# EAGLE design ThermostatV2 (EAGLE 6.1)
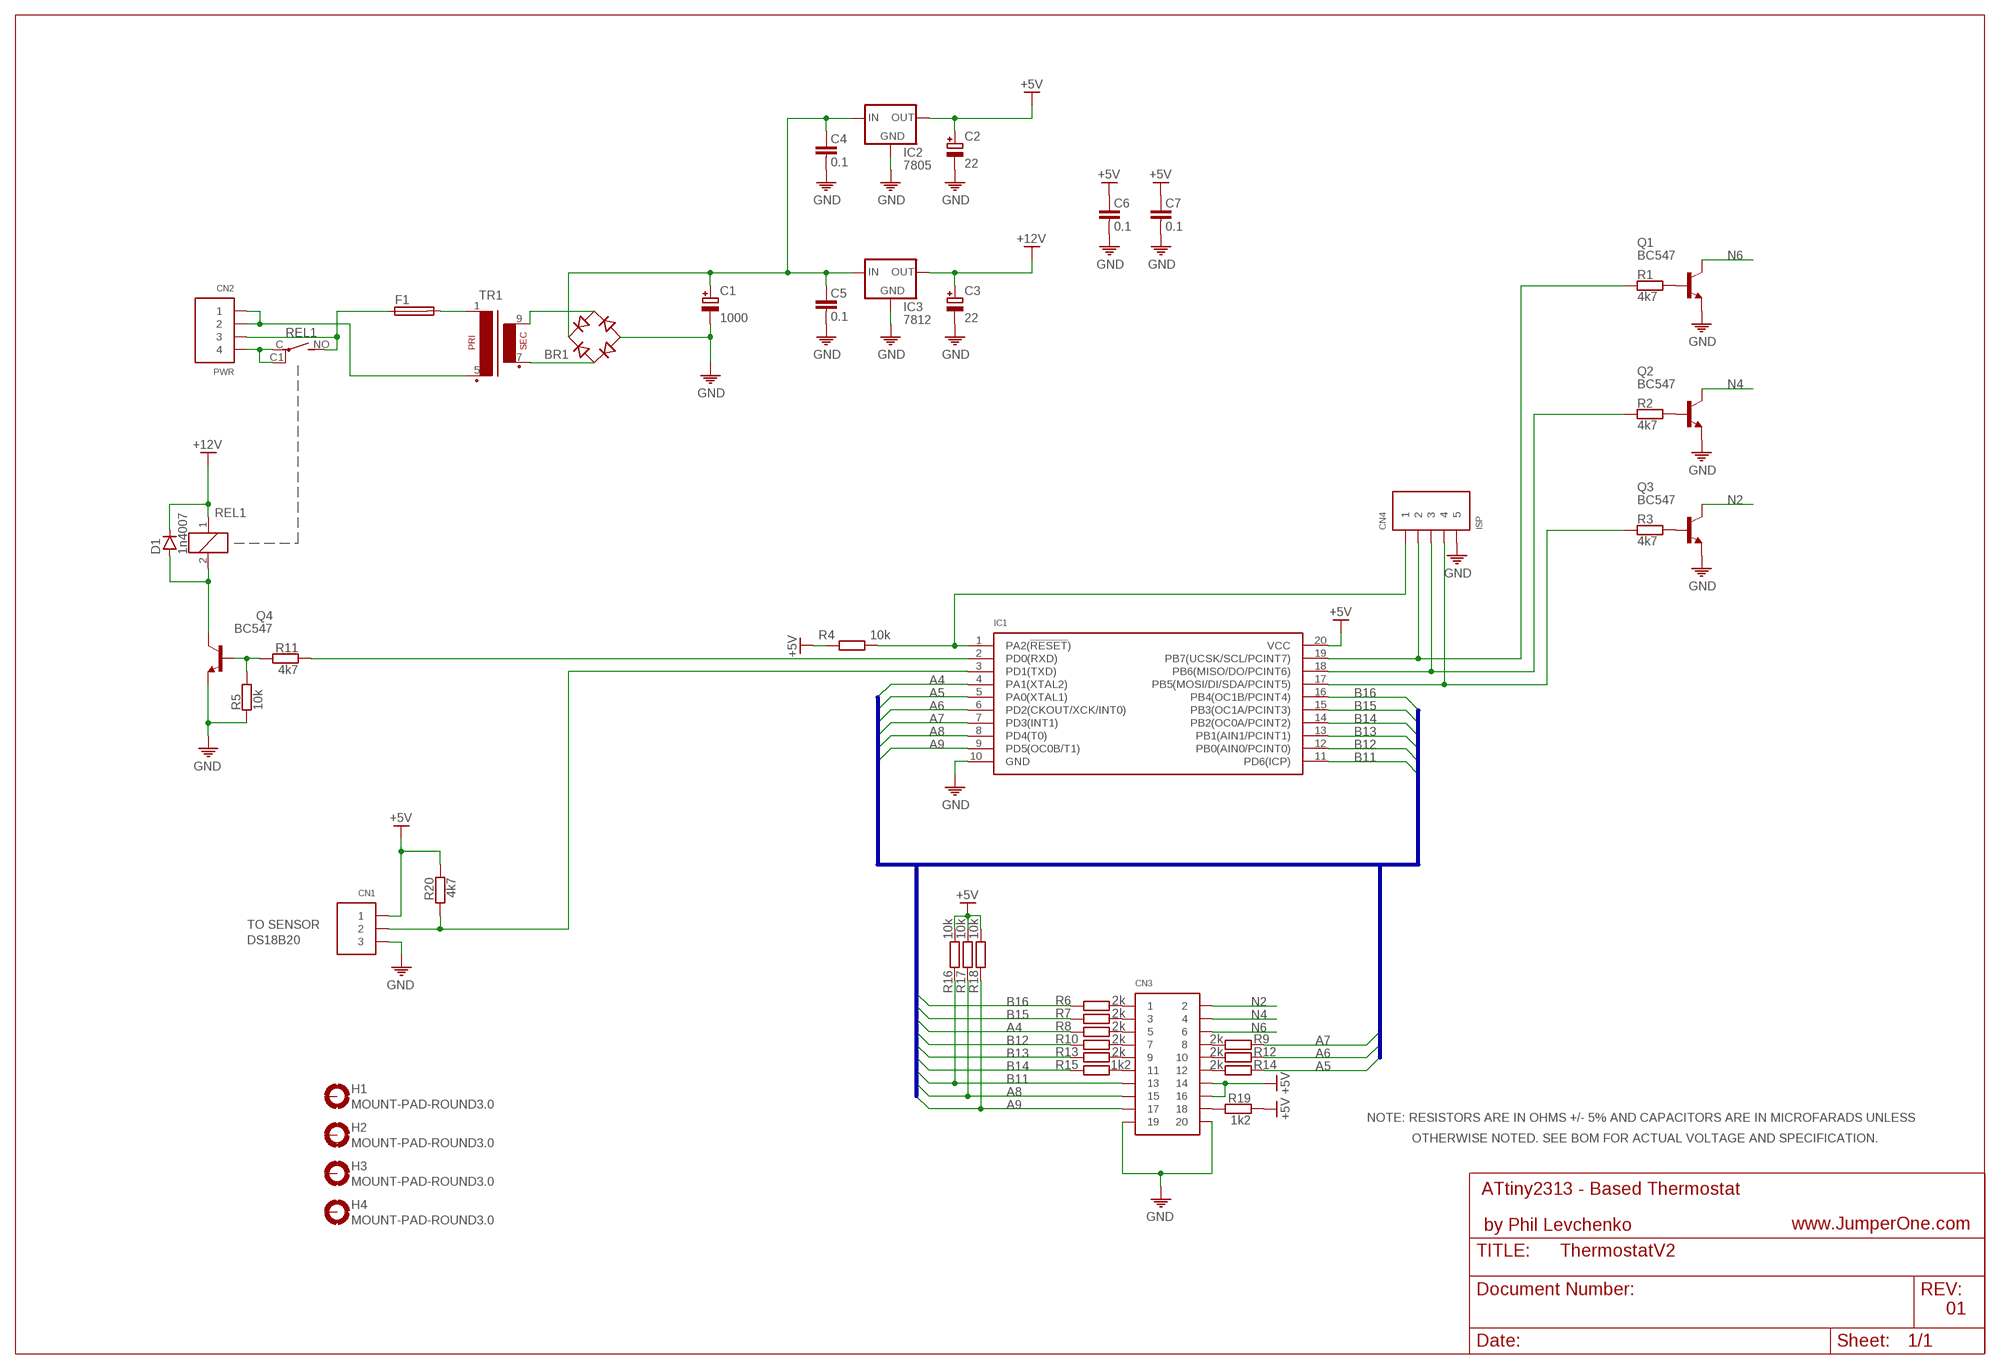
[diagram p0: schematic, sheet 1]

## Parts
BR1  BREC1-DB107  [BREC-DB107]
C1  1000  CPOL-E5-14  [CE5-14]
C2  22  CPOL-E2.5-5  [CE2.5-5]
C3  22  CPOL-E2.5-5  [CE2.5-5]
C4  0.1  C-C050-024X044  [C050-024X044]
C5  0.1  C-C050-024X044  [C050-024X044]
C6  0.1  C-C050-024X044  [C050-024X044]
C7  0.1  C-C050-024X044  [C050-024X044]
CN1  CON-1X03-SCREW-5MM  [CON-SCREW-1X03]
CN2  PWR  CON-1X04-DEGSON-DG25C-B-04P-13  [CON-DEGSON-DG25C-B-04P-13]
CN3  CON-2X10-PH  [CON-PH-2X10]
CN4  ISP  CON-1X05-PH  [CON-PH-1X05]
D1  1n4007  DIODE-DO41-7  [DO41-7]
F1  FUSE-SHK20L  [FUSE-SHK20L]
H1  MOUNT-PAD-ROUND3.0  [3,0-PAD]
H2  MOUNT-PAD-ROUND3.0  [3,0-PAD]
H3  MOUNT-PAD-ROUND3.0  [3,0-PAD]
H4  MOUNT-PAD-ROUND3.0  [3,0-PAD]
IC1  ATMEL-ATTINY2313-DIL20  [DIL20]
IC2  7805  VREG-78XX-TO220-H  [TO-220H]
IC3  7812  VREG-78XX-TO220-H  [TO-220H]
Q1  BC547  TNPN-2N4401-TO92LINE  [TO92-LINE]
Q2  BC547  TNPN-2N4401-TO92LINE  [TO92-LINE]
Q3  BC547  TNPN-2N4401-TO92LINE  [TO92-LINE]
Q4  BC547  TNPN-2N4401-TO92LINE  [TO92-LINE]
R1  4k7  R-AXIAL-0207/7  [R0207-7]
R2  4k7  R-AXIAL-0207/7  [R0207-7]
R3  4k7  R-AXIAL-0207/7  [R0207-7]
R4  10k  R-AXIAL-0207/7  [R0207-7]
R5  10k  R-AXIAL-0207/7  [R0207-7]
R6  2k  R-AXIAL-0207/7  [R0207-7]
R7  2k  R-AXIAL-0207/7  [R0207-7]
R8  2k  R-AXIAL-0207/7  [R0207-7]
R9  2k  R-AXIAL-0207/7  [R0207-7]
R10  2k  R-AXIAL-0207/7  [R0207-7]
R11  4k7  R-AXIAL-0207/7  [R0207-7]
R12  2k  R-AXIAL-0207/7  [R0207-7]
R13  2k  R-AXIAL-0207/7  [R0207-7]
R14  2k  R-AXIAL-0207/7  [R0207-7]
R15  1k2  R-AXIAL-0207/7  [R0207-7]
R16  10k  R-AXIAL-0207/7  [R0207-7]
R17  10k  R-AXIAL-0207/7  [R0207-7]
R18  10k  R-AXIAL-0207/7  [R0207-7]
R19  1k2  R-AXIAL-0207/7  [R0207-7]
R20  4k7  R-AXIAL-0207/7  [R0207-7]
REL1  RELAY-BS-901A  [RELAY-BS901A]
TR1  TRAFO-STEP-DOWN-1P1S-V1  [TRAFO-EI30-1]

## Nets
+5V: C2.+ C6.1 C7.1 CN1.1 CN3.14 CN3.16 IC1.20(VCC) IC2.3(OUT) R4.1 R16.2 R17.2 R18.2 R19.1 R20.1
+12V: C3.+ D1.C IC3.3(OUT) REL1.1
A4: IC1.4(PA1(XTAL2)) R8.1
A5: IC1.5(PA0(XTAL1)) R14.2
A6: IC1.6(PD2(CKOUT/XCK/INT0)) R12.2
A7: IC1.7(PD3(INT1)) R9.2
A8: CN3.15 IC1.8(PD4(T0)) R17.1
A9: CN3.17 IC1.9(PD5(OC0B/T1)) R18.1
B11: CN3.13 IC1.11(PD6(ICP)) R16.1
B12: IC1.12(PB0(AIN0/PCINT0)) R10.1
B13: IC1.13(PB1(AIN1/PCINT1)) R13.1
B14: IC1.14(PB2(OC0A/PCINT2)) R15.1
B15: IC1.15(PB3(OC1A/PCINT3)) R7.1
B16: IC1.16(PB4(OC1B/PCINT4)) R6.1
DS18B20: CN1.2 IC1.3(PD1(TXD)) R20.2
GND: BR1.- C1.- C2.- C3.- C4.2 C5.2 C6.2 C7.2 CN1.3 CN3.19 CN3.20 CN4.5 IC1.10(GND) IC2.2(GND) IC3.2(GND) Q1.3(E) Q2.3(E) Q3.3(E) Q4.3(E) R5.1
N2: CN3.2 Q3.1(C)
N4: CN3.4 Q2.1(C)
N6: CN3.6 Q1.1(C)
N$1: F1.2A TR1.1
N$2: BR1.AC1 TR1.7(S1)
N$3: BR1.AC2 TR1.9(S2)
N$4: CN4.1 IC1.1(PA2(!RESET!)) R4.2
N$5: BR1.+ C1.+ C4.1 C5.1 IC2.1(IN) IC3.1(IN)
N$6: Q1.2(B) R1.2
N$7: Q2.2(B) R2.2
N$8: Q3.2(B) R3.2
N$9: CN4.2 IC1.19(PB7(UCSK/SCL/PCINT7)) R1.1
N$10: CN4.3 IC1.18(PB6(MISO/DO/PCINT6)) R2.1
N$11: CN4.4 IC1.17(PB5(MOSI/DI/SDA/PCINT5)) R3.1
N$12: CN3.1 R6.2
N$13: CN3.3 R7.2
N$14: CN3.5 R8.2
N$15: CN3.8 R9.1
N$16: CN3.7 R10.2
N$17: CN3.10 R12.1
N$18: CN2.3 F1.1A REL1.NO
N$19: CN2.4 REL1.C REL1.C1
N$20: CN2.1 CN2.2 TR1.5(P2)
N$21: D1.A Q4.1(C) REL1.2
N$22: CN3.9 R13.2
N$23: Q4.2(B) R5.2 R11.2
N$24: CN3.12 R14.1
N$25: CN3.11 R15.2
N$26: CN3.18 R19.2
RELAY: IC1.2(PD0(RXD)) R11.1
Unconnected: F1.1B F1.2B H1.B3,0(MOUNT) H2.B3,0(MOUNT) H3.B3,0(MOUNT) H4.B3,0(MOUNT)

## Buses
DBUS:A[2..9],B[11..16]

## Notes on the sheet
- TO SENSOR
- DS18B20
- NOTE: RESISTORS ARE IN OHMS +/- 5% AND CAPACITORS ARE IN MICROFARADS UNLESS
- OTHERWISE NOTED. SEE BOM FOR ACTUAL VOLTAGE AND SPECIFICATION.
- ATtiny2313 - Based Thermostat
- by Phil Levchenko | www.JumperOne.com
- 01

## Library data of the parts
BR1 = JumperOne:BREC1
C1-C3 = JumperOne:CPOL
C4-C7 = JumperOne:C
CN1 = JumperOne:CON-1X03
CN2 = JumperOne:CON-1X04
CN3 = JumperOne:CON-2X10
CN4 = JumperOne:CON-1X05
D1 = JumperOne:DIODE: Silicon Diode
F1 = JumperOne:FUSE
H1-H4 = holes:MOUNT-PAD-ROUND: MOUNTING PAD, round
IC1 = JumperOne:ATMEL-ATTINY2313
IC2 IC3 = JumperOne:VREG-78XX-TO220
Q1-Q4 = JumperOne:TNPN-2N4401: 40V 600mA general purpose switching transistor
R1-R20 = JumperOne:R-AXIAL
REL1 = JumperOne:RELAY-BS-901A
TR1 = JumperOne:TRAFO-STEP-DOWN-1P1S

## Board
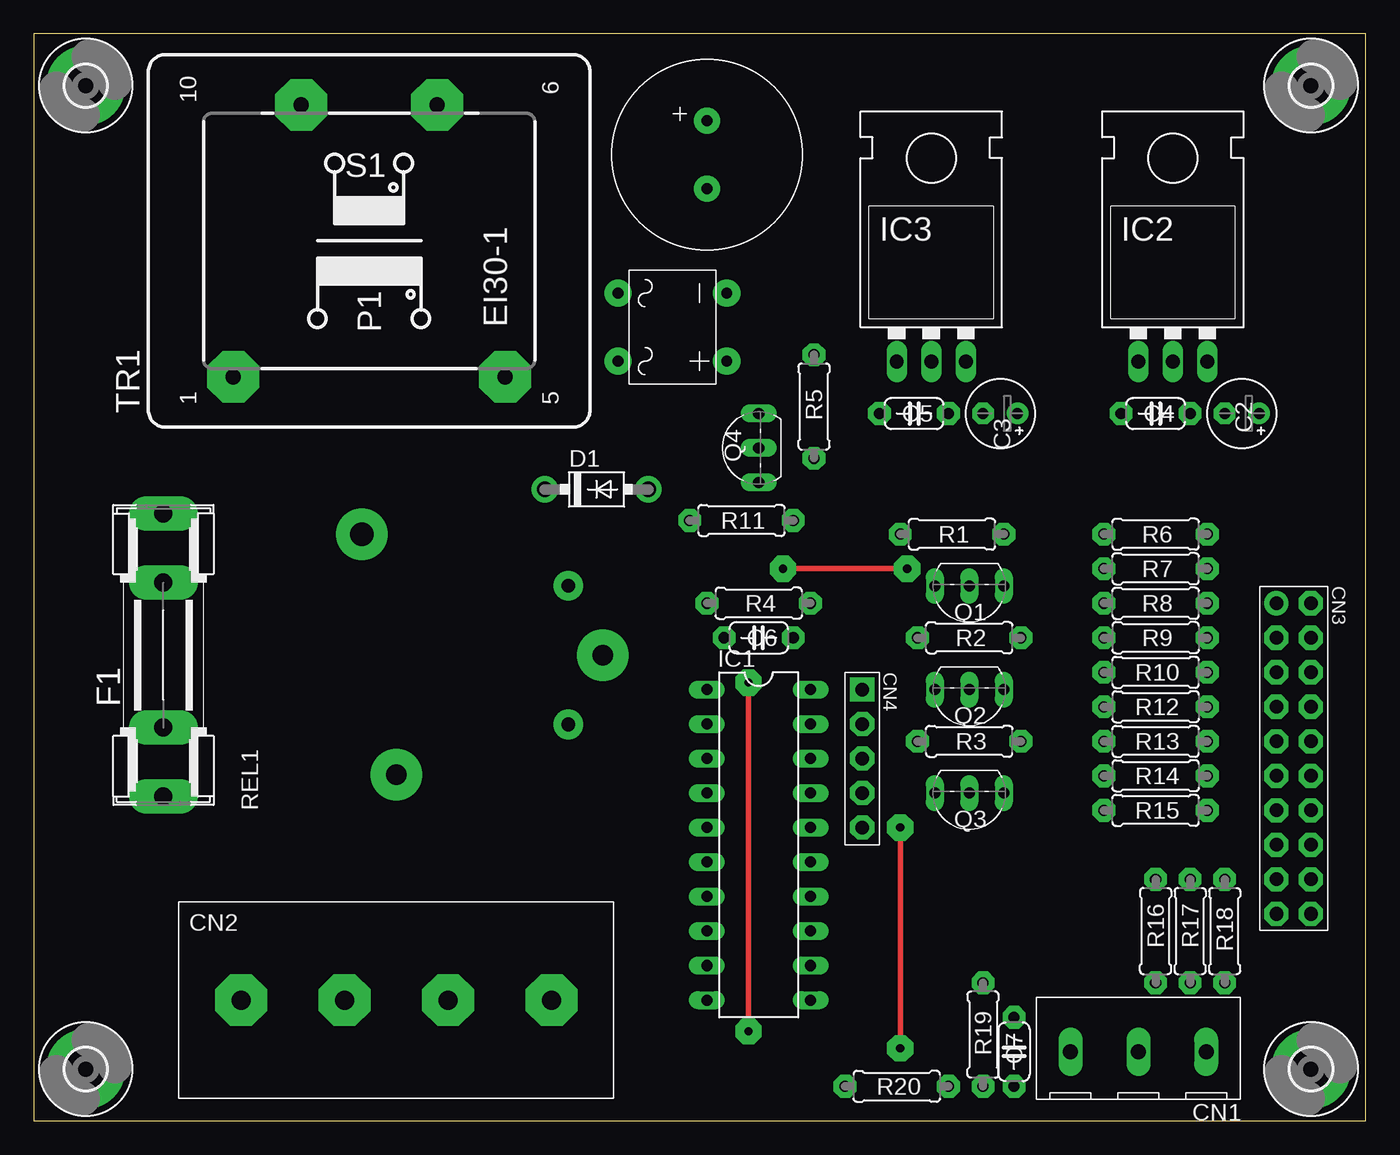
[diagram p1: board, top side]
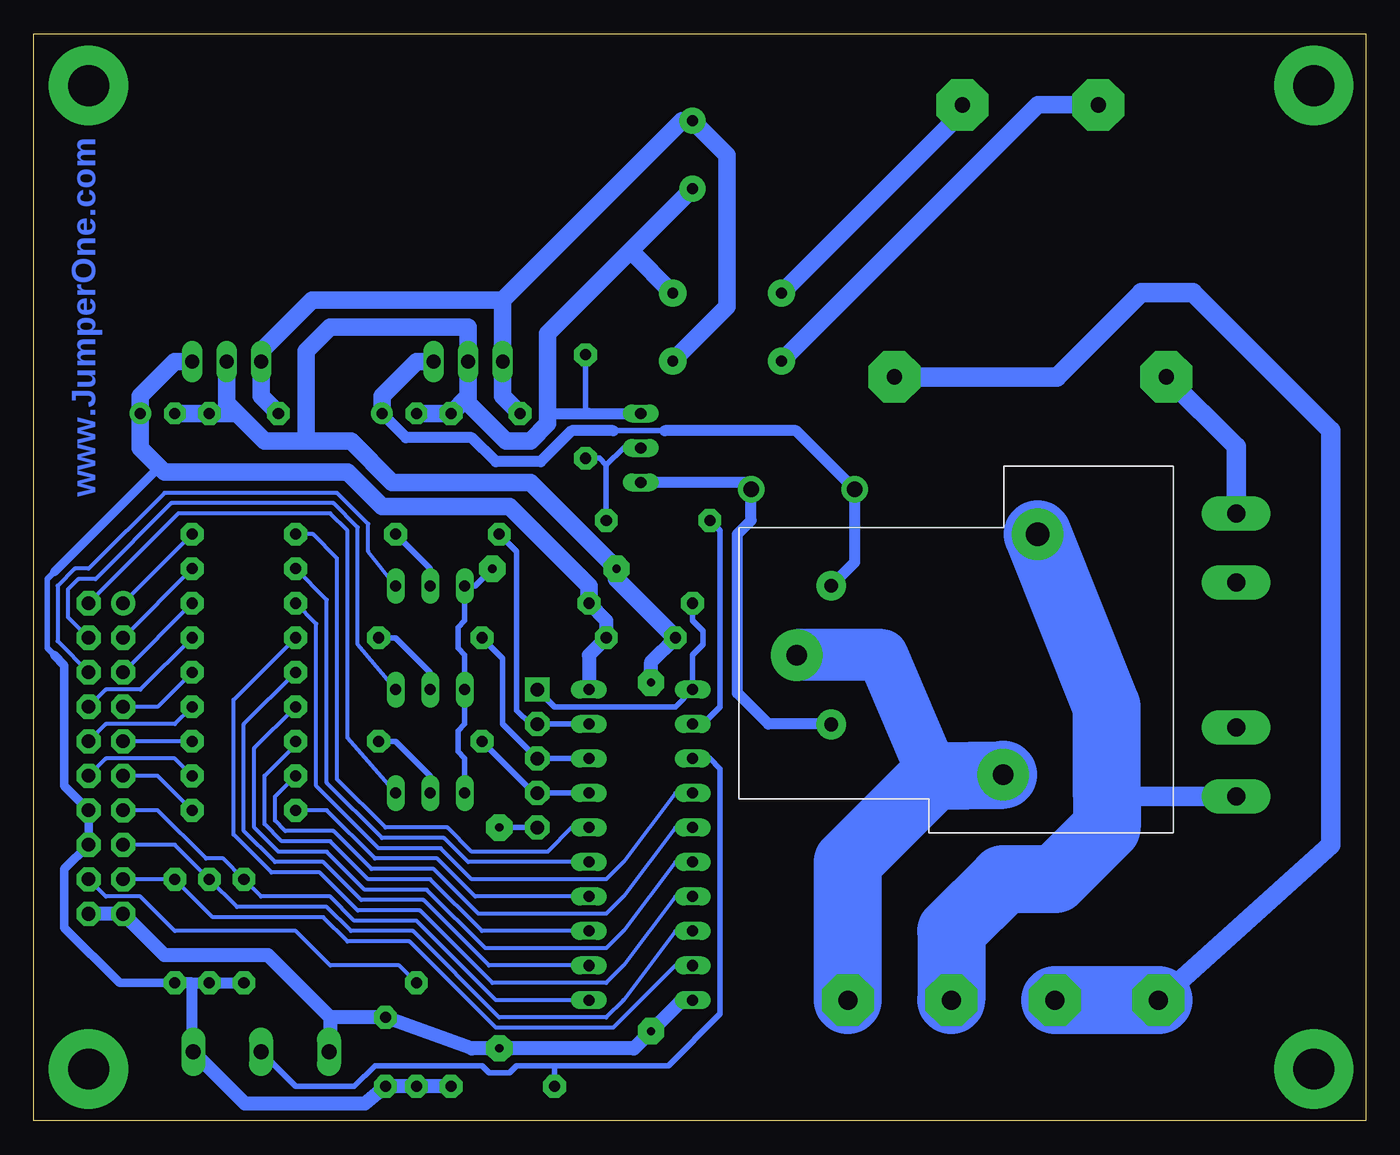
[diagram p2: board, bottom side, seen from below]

Size 98 x 80 mm. Coordinates in mm from the lower left corner, seen from the top.
Outline: 0,0 98,0 98,80 0,80 0,0
Copper layers (1*16): Top 0.035mm / dielectric 1.5mm / Bottom 0.035mm
Design rules: minimum track width 10mil, minimum drill 24mil, track to track 8mil, track to pad 8mil, pad to pad 8mil, via to via 8mil, smd to smd 8mil, copper to edge 40mil, drill to drill 8mil, minimum pad ring 10mil, minimum via ring 8mil, stop-mask expansion 4mil, vias tented up to drill 0mil, thermal gap 10mil

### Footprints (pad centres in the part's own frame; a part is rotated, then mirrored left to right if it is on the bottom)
BREC-DB107 = drill 0.8 pad 2: + 2.5,4; - -2.5,4; AC1 -2.5,-4; AC2 2.5,-4
CE5-14 = drill 0.8 pad 1.93: + 2.5,0; - -2.5,0
CE2.5-5 = drill 0.813 pad 1.6: + -1.27,0 | drill 0.813 pad 1.6 octagon: - 1.27,0
C050-024X044 = drill 0.813 pad 1.676 octagon: 1 -2.54,0; 2 2.54,0
CON-SCREW-1X03 = drill 1.1 pad 1.778 long: 1 -5,0; 2 0,0; 3 5,0
CON-DEGSON-DG25C-B-04P-13 = drill 1.4 pad 3.81 octagon: 1 -11.43,0; 2 -3.81,0; 3 3.81,0; 4 11.43,0
CON-PH-2X10 = drill 1 pad 1.778: 1 -1.27,11.43 | drill 1 pad 1.778 octagon: 2 1.27,11.43; 3 -1.27,8.89; 4 1.27,8.89; 5 -1.27,6.35; 6 1.27,6.35; 7 -1.27,3.81; 8 1.27,3.81; 9 -1.27,1.27; 10 1.27,1.27; 11 -1.27,-1.27; 12 1.27,-1.27; 13 -1.27,-3.81; 14 1.27,-3.81; 15 -1.27,-6.35; 16 1.27,-6.35; 17 -1.27,-8.89; 18 1.27,-8.89; 19 -1.27,-11.43; 20 1.27,-11.43
CON-PH-1X05 = drill 1 pad 1.778 square: 1 0,5.08 | drill 1 pad 1.778 octagon: 2 0,2.54; 3 0,0; 4 0,-2.54; 5 0,-5.08
DO41-7 = drill 1.118 pad 1.93: A 3.81,0; C -3.81,0
FUSE-SHK20L = drill 1.321 pad 2.54 long: 1A -10.414,0; 1B -5.334,0; 2A 10.414,0; 2B 5.334,0
3,0-PAD = drill 3 pad 5.842: B3,0 0,0
DIL20 = drill 0.813 long: 1 -11.43,-3.81; 2 -8.89,-3.81; 3 -6.35,-3.81; 4 -3.81,-3.81; 5 -1.27,-3.81; 6 1.27,-3.81; 7 3.81,-3.81; 8 6.35,-3.81; 9 8.89,-3.81; 10 11.43,-3.81; 11 11.43,3.81; 12 8.89,3.81; 13 6.35,3.81; 14 3.81,3.81; 15 1.27,3.81; 16 -1.27,3.81; 17 -3.81,3.81; 18 -6.35,3.81; 19 -8.89,3.81; 20 -11.43,3.81
TO-220H = drill 1.016 long: 1 -2.54,-8.89; 2 0,-8.89; 3 2.54,-8.89
TO92-LINE = drill 0.813 long: 1 -2.54,0; 2 0,0; 3 2.54,0
R0207-7 = drill 0.813 pad 1.676 octagon: 1 -3.81,0; 2 3.81,0
RELAY-BS901A = drill 1 pad 2.184: 1 5.09,-10.12; 2 -5.11,-10.12 | drill 1.5 pad 3.81: C -8.81,2.54; C1 -0.01,-12.66 | drill 1.7 pad 3.81: NO 8.89,5.08
TRAFO-EI30-1 = drill 1.118 pad 3.81 octagon: 1 -10.008,10.008; 5 -10.008,-10.008; 7 10.008,-5.004; 9 10.008,5.004

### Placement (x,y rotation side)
BR1  46.99,58.42 270 top
C1  49.53,71.12 90 top
C2  88.9,52.07 180 top
C3  71.12,52.07 180 top
C4  82.55,52.07 0 top
C5  64.77,52.07 0 top
C6  53.34,35.56 180 top
C7  72.14,5.08 90 top
CN1  81.28,5.08 180 top
CN2  26.67,8.89 0 top
CN3  92.71,26.67 0 top
CN4  60.96,26.67 0 top
D1  41.4,46.48 0 top
F1  9.53,34.29 90 top
H1  93.98,76.2 0 top
H2  93.98,3.81 0 top
H3  3.81,76.2 0 top
H4  3.81,3.81 0 top
IC1  53.34,20.32 270 top
IC2  83.82,64.77 0 top
IC3  66.04,64.77 0 top
Q1  68.83,39.37 180 top
Q2  68.83,31.75 180 top
Q3  68.83,24.13 180 top
Q4  53.34,49.53 90 top
R1  67.56,43.18 0 top
R2  68.83,35.56 0 top
R3  68.83,27.94 0 top
R4  53.34,38.1 180 top
R5  57.4,52.58 270 top
R6  82.55,43.18 0 top
R7  82.55,40.64 0 top
R8  82.55,38.1 0 top
R9  82.55,35.56 180 top
R10  82.55,33.02 0 top
R11  52.07,44.2 0 top
R12  82.55,30.48 180 top
R13  82.55,27.94 0 top
R14  82.55,25.4 180 top
R15  82.55,22.86 0 top
R16  82.55,13.97 270 top
R17  85.09,13.97 270 top
R18  87.63,13.97 270 top
R19  69.85,6.35 90 top
R20  63.5,2.54 180 top
REL1  29.21,34.29 90 top
TR1  24.67,64.77 90 top

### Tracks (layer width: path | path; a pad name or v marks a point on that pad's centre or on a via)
+5V
  Bottom 0.406: 96.52,34.29 97.03,34.8 97.03,39.88 96.52,40.39
  Bottom 0.61: R18.2 91.69,10.16 95.76,14.22 95.76,18.54 CN3.16 CN3.14 95.76,24.64 95.76,33.53 96.52,34.29 | 96.52,40.39 88.77,48.13
  Bottom 0.813: R16.2 R17.2 86.36,10.16 | 86.36,10.16 R18.2 | CN1.1 86.36,5.16 86.36,10.16
  Bottom 1.016: IC1.20 57.15,34.29 C6.1 55.88,36.83 R4.1 | CN1.1 82.47,1.27 73.66,1.27 C7.1 R19.1 R20.1
  Bottom 1.27: IC2.3 87.63,55.88 90.17,53.34 C2.+ 90.17,49.53 88.77,48.13 88.39,47.75 74.93,47.75 72.39,45.21 62.99,45.21 57.15,39.37 R4.1
+12V
  Bottom 0.406: 51.56,50.8 55.37,50.8
  Bottom 0.813: C3.+ 70.61,50.29 65.79,50.29 64.01,48.51 60.71,48.51 58.42,50.8 55.37,50.8 | 51.56,50.8 41.91,50.8 D1.C 37.59,41.12 REL1.1
  Bottom 1.27: IC3.3 69.85,55.88 72.39,53.34 C3.+
A4
  Bottom 0.305: R8.1 77.22,36.58 77.22,24.64 72.64,20.07 68.07,20.07 65.79,17.78 55.88,17.78 54.61,19.05 50.8,24.13 IC1.4
A5
  Bottom 0.305: R14.2 80.26,23.88 80.26,22.1 79.5,21.34 75.95,21.34 73.15,18.54 68.58,18.54 65.28,15.24 55.88,15.24 54.61,16.51 50.8,21.59 IC1.5
A6
  Bottom 0.305: R12.2 81.79,27.43 81.79,21.59 80.01,19.81 76.45,19.81 73.66,17.02 69.09,17.02 64.77,12.7 55.88,12.7 54.61,13.97 50.8,19.05 IC1.6
A7
  Bottom 0.305: R9.2 83.31,30.99 83.31,21.08 80.52,18.29 76.96,18.29 74.17,15.49 69.6,15.49 64.26,10.16 55.88,10.16 54.61,11.43 50.8,16.51 IC1.7
A8
  Bottom 0.305: CN3.15 87.63,20.32 R17.1 83.06,15.75 76.45,15.75 74.68,13.97 70.1,13.97 63.75,7.62 55.88,7.62 54.61,8.89 50.8,13.97 IC1.8
A9
  Bottom 0.305: CN3.17 R18.1 84.84,14.99 76.71,14.99 74.93,13.21 70.36,13.21 64.01,6.86 55.37,6.86 50.8,11.43 IC1.9
B11
  Bottom 0.305: CN3.13 88.9,22.86 85.34,19.3 84.07,19.3 R16.1 81.28,16.51 76.2,16.51 74.42,14.73 69.85,14.73 64.01,8.89 IC1.11
B12
  Bottom 0.305: R10.1 82.55,29.21 82.55,21.34 80.26,19.05 76.71,19.05 73.91,16.26 69.34,16.26 64.52,11.43 IC1.12
B13
  Bottom 0.305: 78.74,27.69 81.03,25.4 81.03,21.84 79.76,20.57 76.2,20.57 73.41,17.78 68.83,17.78 65.02,13.97 IC1.13
  Bottom 0.406: 78.74,27.69 R13.1
B14
  Bottom 0.305: R15.1 76.45,22.86 72.9,19.3 68.33,19.3 65.53,16.51 IC1.14
B15
  Bottom 0.305: R7.1 76.45,38.35 76.45,24.89 72.39,20.83 67.82,20.83 66.04,19.05 IC1.15
B16
  Bottom 0.305: R6.1 77.47,43.18 75.69,41.4 75.69,25.15 72.14,21.59 67.56,21.59 65.79,19.81 60.2,19.81 58.42,21.59 IC1.16
DS18B20
  Bottom 0.406: CN1.2 78.74,2.54 74.42,2.54 72.9,4.06 65.02,4.06 64.52,3.56 62.99,3.56 62.48,4.06 59.69,4.06 | 59.69,4.06 51.31,4.06 47.5,7.87 47.5,25.91 48.26,26.67 IC1.3 | 59.69,4.06 R20.2
GND  (via drill 0.6 pad 1.93)
  Top 0.406: v63.75,5.33 v63.75,21.59 | v55.12,40.64 v64.26,40.64 | v52.58,6.6 v52.58,32.26
  Bottom 0.406: Q3.3 66.29,26.67 66.8,27.18 66.8,28.7 66.29,29.21 Q2.3 66.29,34.29 66.8,34.8 66.8,36.32 66.29,36.83 Q1.3 65.53,39.37 v64.26,40.64 | v63.75,21.59 CN4.5 | R5.1 57.4,52.32 57.15,52.07
  Bottom 0.813: 60.2,51.31 60.2,52.07 57.15,52.07 Q4.3
  Bottom 1.016: 66.04,53.85 66.04,53.34 | IC1.10 50.29,8.89 v52.58,6.6 53.85,5.33 v63.75,5.33 65.79,5.33 C7.2 76.2,7.62 | C6.2 52.58,33.78 v52.58,32.26 | CN3.20 CN3.19 88.39,12.19 80.77,12.19 76.2,7.62 | CN1.3 76.2,5.08 76.2,7.62
  Bottom 1.27: 66.04,53.34 C5.2 C3.- | C2.- C4.2 83.06,52.07 | 53.99,64.16 60.2,57.95 60.2,51.31 61.47,50.04 63.25,50.04 66.04,52.83 66.04,53.85 IC3.2 66.04,58.42 76.2,58.42 77.98,56.64 77.98,50.04 | 53.99,64.16 C1.- | 77.98,50.04 81.03,50.04 83.06,52.07 | IC2.2 83.82,52.83 83.06,52.07 | 77.98,50.04 74.68,50.04 71.63,46.99 61.47,46.99 v55.12,40.64 55.12,39.88 C6.2 | BR1.- 53.99,63.92 53.99,64.16
N2
  Bottom 0.305: Q3.1 74.93,28.19 74.93,43.43 76.2,44.7 87.38,44.7 CN3.2
N4
  Bottom 0.305: Q2.1 74.17,35.05 74.17,43.69 75.95,45.47 87.88,45.47 93.47,39.88 94.74,39.88 95.5,39.12 95.5,37.08 CN3.4
N6
  Bottom 0.305: Q1.1 73.41,41.91 73.41,43.94 75.69,46.23 88.39,46.23 93.98,40.64 95,40.64 96.27,39.37 96.27,35.31 CN3.6
N$1
  Bottom 1.422: F1.2A 9.53,49.62 TR1.1
N$2
  Bottom 1.27: BR1.AC1 29.67,74.24 TR1.7
N$3
  Bottom 1.27: TR1.9 24.13,74.78 BR1.AC2
N$4
  Bottom 0.406: R4.2 49.53,36.83 48.77,36.07 48.77,35.05 49.53,34.29 IC1.1 50.8,30.48 59.69,30.48 CN4.1
N$5
  Bottom 1.27: C5.1 63.5,53.34 IC3.1 63.5,60.41 | C4.1 81.28,53.34 IC2.1 81.28,56.64 77.51,60.41 63.5,60.41 | 63.5,60.41 50.29,73.62 C1.+ 46.99,71.08 46.99,59.92 BR1.+
N$6
  Bottom 0.406: Q1.2 68.83,40.64 R1.2
N$7
  Bottom 0.406: Q2.2 68.83,33.02 71.37,35.56 R2.2
N$8
  Bottom 0.406: Q3.2 68.83,25.4 71.37,27.94 R3.2
N$9
  Bottom 0.406: IC1.19 CN4.2 61.47,29.21 62.48,30.23 62.48,41.91 R1.1
N$10
  Bottom 0.406: IC1.18 CN4.3 63.5,29.21 63.5,34.04 R2.1
N$11
  Bottom 0.406: IC1.17 CN4.4 61.21,24.13 R3.1
N$12
  Bottom 0.305: R6.2 CN3.1
N$13
  Bottom 0.305: R7.2 CN3.3
N$14
  Bottom 0.305: R8.2 CN3.5
N$15
  Bottom 0.305: R9.1 90.17,31.75 92.71,31.75 CN3.8
N$16
  Bottom 0.305: R10.2 88.9,30.48 CN3.7
N$17
  Bottom 0.305: R12.1 87.63,29.21 92.71,29.21 CN3.10
N$18
  Bottom 1.422: F1.1A 18.8,23.88 arc90 19.05,24.13
  Bottom 5: CN2.3 30.48,13.97 26.67,17.78 22.86,17.78 19.05,21.59 19.05,24.13 19.05,30.48 REL1.NO
N$19
  Bottom 3.81: REL1.C1 35.56,34.29 31.75,25.4
  Bottom 5: CN2.4 38.1,19.05 31.75,25.4 REL1.C
N$20
  Bottom 1.422: TR1.5 22.71,54.76 16.51,60.96 12.7,60.96 2.54,50.8 2.54,20.32 CN2.1
  Bottom 5: CN2.1 CN2.2
N$21
  Bottom 0.813: Q4.1 45.72,46.99 D1.A 45.21,44.2 46.23,43.18 46.23,31.5 43.94,29.21 39.36,29.21 REL1.2
N$22
  Bottom 0.305: R13.2 CN3.9
N$23
  Bottom 0.406: R11.2 55.88,48.26 | 55.88,48.26 54.61,49.53 Q4.2 | R5.2 56.39,48.77 55.88,48.26
N$24
  Bottom 0.305: R14.1 87.63,26.67 92.71,26.67 CN3.12
N$25
  Bottom 0.305: R15.2 88.9,25.4 CN3.11
N$26
  Bottom 0.305: R19.2 71.12,11.43 76.2,11.43 78.74,13.97 87.63,13.97 90.17,16.51 92.71,16.51 CN3.18
RELAY
  Bottom 0.406: R11.1 47.5,43.43 47.5,30.48 48.77,29.21 IC1.2

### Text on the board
Bottom: www.JumperOne.com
